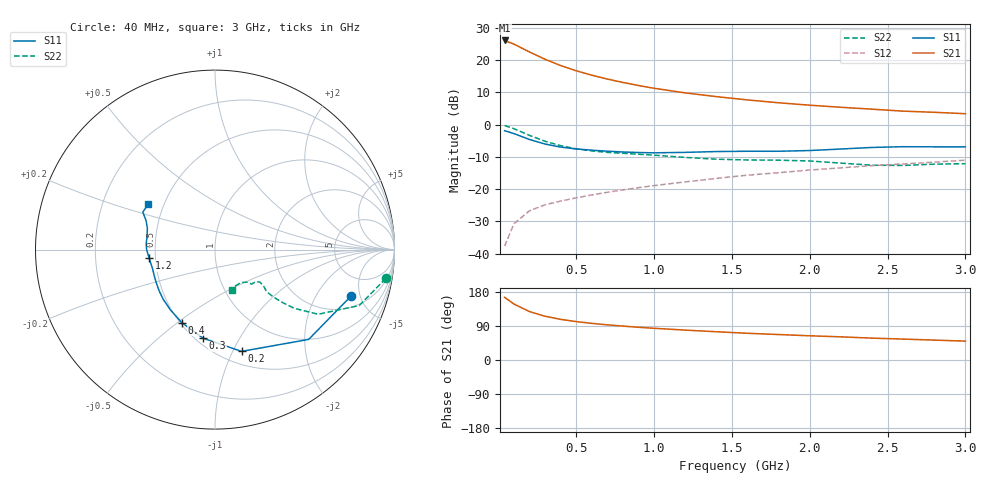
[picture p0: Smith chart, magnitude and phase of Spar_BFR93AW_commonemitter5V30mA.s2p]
! Filename:  BFR93AWD.S2P  Version:  4.0
! NXP part #: BFR93AW  Date: Jun 1994
! Bias condition: Vce=5V, Ic=30mA
#  MHz  S  MA  R  50
! Freq  S11  S21  S12  S22  !GUM [dB]
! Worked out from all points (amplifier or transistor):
!   21 points, 40 MHz to 3 GHz, reference 50 ohm
!   highest |S21| = 26.1 dB at 40 MHz (marker M1)
!   |S21| within 3 dB of that: start of sweep to 176.4 MHz
!   unconditionally stable (mu >= 1): 932.2 MHz to end of sweep
!   at 300 MHz: K = 0.58, MSG = 22.6 dB, |S12| = -24.9 dB
!   at 1 GHz: K = 1.02, MAG = 14.2 dB, |S12| = -18.9 dB
!   at 3 GHz: K = 1.03, MAG = 6.2 dB, |S12| = -11.1 dB
!   lowest NFmin = 2.10 dB at 500 MHz
!   S11 on the Smith chart (normalised r, x): 40 MHz: 2.88, -4.15; 200 MHz: 0.63, -1.08; 300 MHz: 0.54, -0.71; 400 MHz: 0.51, -0.52; 1.2 GHz: 0.46, -0.05; 3 GHz: 0.41, +0.26
40  0.802 -18.7  20.1 165.4  0.013 80.4  0.965 -9.6
100  0.723 -43.8  17.62 147.7  0.029 69.4  0.862 -21.2
200  0.586 -75.4  13.32 127.7  0.046 59.6  0.678 -32.1
300  0.498 -97.7  10.26 115.4  0.057 56.0  0.55 -36.5
400  0.447 -114.4  8.211 107.2  0.065 55.9  0.47 -38.3
500  0.418 -126.4  6.807 101.3  0.073 56.8  0.42 -39.0
600  0.4 -136.2  5.817 96.7  0.081 58.4  0.39 -39.2
700  0.386 -144.1  5.066 92.8  0.089 59.9  0.37 -38.9
800  0.375 -151.1  4.487 89.5  0.097 61.2  0.358 -38.4
900  0.368 -157.2  4.025 86.3  0.105 62.4  0.346 -37.4
1000  0.364 -163.0  3.648 83.7  0.113 63.5  0.335 -36.7
1200  0.37 -172.8  3.092 78.9  0.129 65.2  0.309 -35.9
1400  0.381 -179.9  2.708 74.6  0.146 66.5  0.29 -38.0
1600  0.385 174.7  2.406 70.5  0.164 66.9  0.282 -41.8
1800  0.385 169.1  2.173 67.2  0.179 67.8  0.28 -43.5
2000  0.395 162.5  1.993 63.9  0.197 68.5  0.272 -43.9
2200  0.417 157.1  1.851 61.1  0.213 69.0  0.252 -45.8
2400  0.441 154.0  1.729 57.7  0.23 69.2  0.234 -52.0
2600  0.453 152.5  1.612 55.2  0.245 68.9  0.232 -60.1
2800  0.451 149.7  1.547 52.5  0.261 69.2  0.243 -64.9
3000  0.451 145.5  1.471 49.8  0.28 69.1  0.247 -67.3
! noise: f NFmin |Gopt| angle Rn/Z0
500  2.1  0.124  134.7  0.22
1000  2.6  0.233  163.9  0.25
2000  3.4  0.606  -149.3  0.18
